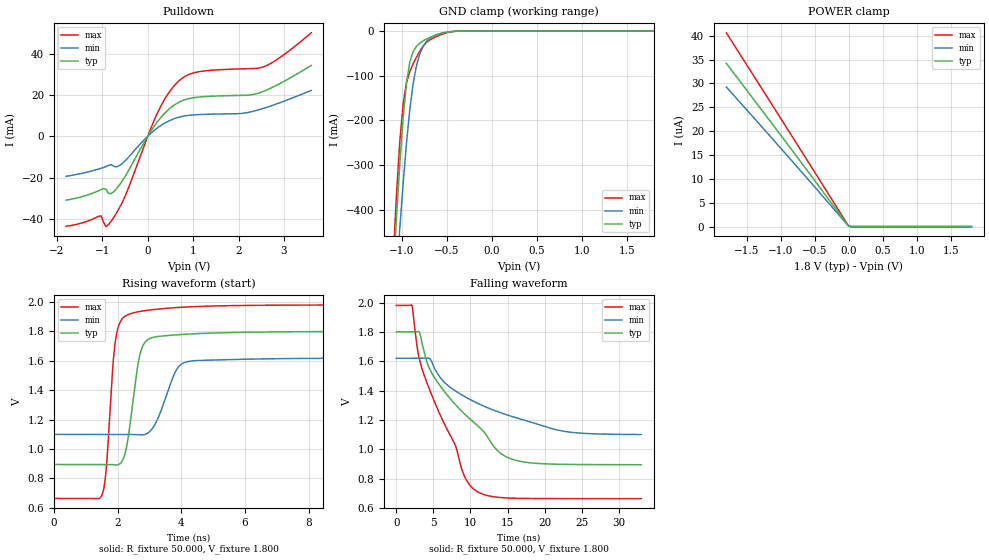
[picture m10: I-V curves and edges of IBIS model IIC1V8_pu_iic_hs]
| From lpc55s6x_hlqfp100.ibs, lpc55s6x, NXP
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|   Model IIC1V8_pu_iic_hs
[Model] IIC1V8_pu_iic_hs
Model_type I/O_open_drain
Polarity   Non-Inverting
Enable   Active-Low
Vinl =  0.540V
Vinh =  1.260V
Vmeas =  0.900V
Cref =  0.0F
Rref =  100.000
Vref =  1.800V
C_comp   2.440pF   2.391pF   2.494pF
C_comp_pulldown   1.723pF   1.659pF   1.780pF
C_comp_power_clamp   0.389pF   0.357pF   0.435pF
[Model Spec]
Vinh   1.260V   1.134V   1.386V
Vinl   0.540V   0.486V   0.594V
Vmeas   0.900V   0.810V   0.990V
Vref   1.800V   1.620V   1.980V
Cref   0.0F   0.0F   0.0F
Rref   100.000   100.000   100.000
[Temperature Range]   25.000   0.125k   -40.000
[Voltage Range]   1.800V   1.620V   1.980V
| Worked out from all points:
|   slope of the pulldown table from 0 to 0.27 V, typ, clamps not added: 31.5 ohm
|   GND clamp passes 1 mA (typ) near -0.44 V on its own axis
|   rising waveform, R_fixture 50.000, V_fixture 1.800: 20-80 % time 347ps typ, 536ps min, 254ps max; typ from 0.895 V to 1.8 V
|   falling waveform, R_fixture 50.000, V_fixture 1.800: 20-80 % time 8.41ns typ, 11.3ns min, 5.73ns max; typ from 1.8 V to 0.896 V
[Pulldown]
|Voltage   I(typ)   I(min)   I(max)
-1.8V     -30.97mA   -19.41mA   -43.61mA
-1.03V    -25.91mA   -15.56mA   -38.59mA
-920mV    -25.75mA   -14.67mA   -43.75mA
-865mV    -27.69mA   -14.16mA   -42.79mA
-700mV    -25.69mA   -14.87mA   -37.58mA
-480mV    -18.8mA    -11.48mA   -28.03mA
235mV     7.619mA    4.356mA    12.23mA
455mV     12.83mA    7.267mA    20.76mA
730mV     16.88mA    9.427mA    27.6mA
1.17V     19mA       10.49mA    31.33mA
2.545V    21.66mA    13.44mA    33.54mA
3.6V      34.22mA    22.14mA    50.01mA
[GND_clamp]
|Voltage   I(typ)   I(min)   I(max)
-1.8V     -3.488A    -3.23A     -3.872A
-1.097V   -545.6mA   -658.5mA   -507.1mA
-1.06V    -414.6mA   -546.1mA   -365.1mA
-1.023V   -294.9mA   -439.1mA   -246mA
-986mV    -192.5mA   -339.6mA   -162mA
-949mV    -115.7mA   -250.4mA   -115.2mA
-912mV    -69.22mA   -175.3mA   -90.67mA
-838mV    -34.06mA   -77.19mA   -58.54mA
-764mV    -21.86mA   -34.13mA   -33.64mA
-653mV    -11.47mA   -11.68mA   -15.87mA
-431mV    -870uA     -906.4uA   -1.185mA
1.8V      0A         0A         0A
[POWER_clamp]
|Voltage   I(typ)   I(min)   I(max)
-1.8V     34.22uA    29.25uA    40.61uA
-864mV    16.54uA    14.2uA     19.57uA
-13mV     251.2nA    223.3nA    296.4nA
24mV      0A         0A         0A
1.8V      0A         0A         0A
[Ramp]
| variable   typ   min   max
dV/dt_r   0.543/0.347n   0.312/0.536n   0.790/0.254n
dV/dt_f   0.543/8.410n   0.311/11.264n   0.789/5.728n
R_load = 50.000
[Rising Waveform]
R_fixture= 50.000
V_fixture= 1.800
V_fixture_min= 1.620
V_fixture_max= 1.980
|time   V(typ)   V(min)   V(max)
0s        895.1mV    1.1V       664.1mV
1.504ns   895.1mV    1.1V       684.6mV
1.64ns    895.2mV    1.1V       854.1mV
1.857ns   894mV      1.1V       1.579V
1.981ns   892.4mV    1.1V       1.795V
2.282ns   1.014V     1.1V       1.91V
2.701ns   1.641V     1.096V     1.936V
3.897ns   1.777V     1.555V     1.963V
4.436ns   1.784V     1.601V     1.969V
33ns      1.8V       1.62V      1.98V
[Falling Waveform]
R_fixture= 50.000
V_fixture= 1.800
V_fixture_min= 1.620
V_fixture_max= 1.980
|time   V(typ)   V(min)   V(max)
0s        1.8V       1.62V      1.98V
2.118ns   1.8V       1.62V      1.98V
2.889ns   1.802V     1.62V      1.675V
3.667ns   1.681V     1.62V      1.519V
5.51ns    1.461V     1.52V      1.281V
7.966ns   1.305V     1.398V     1.027V
9.222ns   1.24V      1.36V      813.4mV
10.5ns    1.181V     1.325V     726.9mV
16.16ns   924.6mV    1.215V     667.1mV
33ns      895.7mV    1.101V     664.3mV
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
